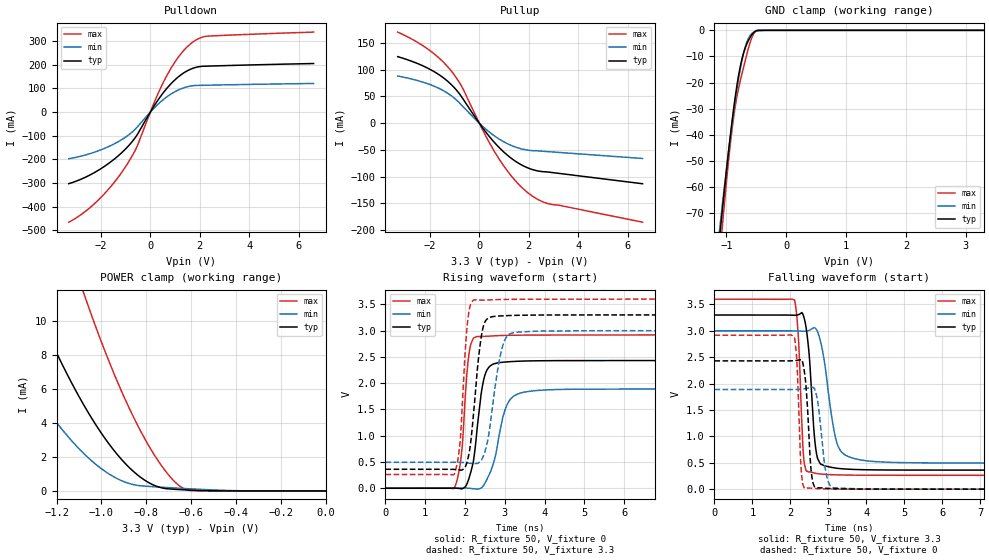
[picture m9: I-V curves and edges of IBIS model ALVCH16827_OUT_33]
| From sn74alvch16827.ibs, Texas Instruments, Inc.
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[Model]   ALVCH16827_OUT_33
Model_type  3-state
Enable   Active-Low
Vref =   0
Rref =   500
Cref =   50p
Vmeas =   1.5
| variable   typ   min   max
C_comp   3.97pF   3.54pF   4.17pF
| C_pullup   5.12pF   4.43pF   5.61pF
| C_pulldown   8.30pF   4.57pF   11.95pF
| C_tri-state   3.97pF   3.54pF   4.17pF
[Temperature Range]   40   100   -40
| Ambient temperature   25   85   -40
[Voltage range]   3.3   3   3.6
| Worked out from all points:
|   slope of the pulldown table from 0 to 0.495 V, typ, clamps not added: 6.36 ohm
|   slope of the pullup table from 0 to 0.495 V, typ, clamps not added: 16.5 ohm
|   GND clamp passes 1 mA (typ) near -0.55 V on its own axis
|   POWER clamp passes 1 mA (typ) near -0.84 V on its own axis
|   rising waveform, R_fixture 50, V_fixture 0: 20-80 % time 235ps typ, 343ps min, 166ps max; typ from 0 V to 2.43 V
|   falling waveform, R_fixture 50, V_fixture 3.3: 20-80 % time 167ps typ, 304ps min, 117ps max; typ from 3.3 V to 0.361 V
|   rising waveform, R_fixture 50, V_fixture 3.3: 20-80 % time 223ps typ, 290ps min, 155ps max; typ from 0.361 V to 3.3 V
|   falling waveform, R_fixture 50, V_fixture 0: 20-80 % time 119ps typ, 174ps min, 90.7ps max; typ from 2.43 V to 0 V
[GND Clamp]
| ALVCH16827_OUT_33
|   Voltage   I(typ)   I(min)   I(max)
-3.3V     -675.5mA   -611.9mA   -772mA
-1.12V    -80.81mA   -77.55mA   -88.84mA
-1.1V     -76.16mA   -73.37mA   -83.51mA
-1.075V   -70.43mA   -68.21mA   -76.96mA
-1.055V   -65.91mA   -64.14mA   -71.81mA
-905mV    -34.72mA   -35.65mA   -37.77mA
-845mV    -24.31mA   -25.69mA   -28.1mA
-780mV    -15.21mA   -16.34mA   -20.53mA
-655mV    -4.986mA   -4.361mA   -8.861mA
-575mV    -1.715mA   -1.195mA   -2.821mA
-510mV    -244.5uA   -419.5uA   -312.1uA
3.3V      1.222nA    1.002uA    51.57pA
[POWER Clamp]
| ALVCH16827_OUT_33
|   Voltage   I(typ)   I(min)   I(max)
-3.3V     106mA      74.09mA    151.6mA
-1.545V   19.46mA    11.49mA    33.45mA
-1.32V    11.68mA    6.284mA    22.02mA
-1.295V   10.9mA     5.78mA     20.85mA
-1.195V   7.991mA    3.942mA    16.37mA
-1.075V   4.975mA    2.155mA    11.49mA
-965mV    2.743mA    987.9uA    7.581mA
-860mV    1.177mA    378.6uA    4.425mA
-760mV    302.3uA    241.6uA    2.031mA
-660mV    86.32uA    163.9uA    380.1uA
-605mV    48.51uA    124.7uA    22.06uA
-48.03fV  1.222nA    59.96nA    62.94pA
[Pulldown]
| ALVCH16827_OUT_33
|   Voltage   I(typ)   I(min)   I(max)
-3.3V     -302.4mA   -196.9mA   -465.1mA
-2.73V    -280.1mA   -184.3mA   -427.4mA
-2.16V    -249.3mA   -165.8mA   -377mA
-1.61V    -210.9mA   -141.8mA   -315.8mA
-1.105V   -166.3mA   -112.9mA   -246.6mA
-565mV    -100.8mA   -67.07mA   -151.3mA
185mV     31.43mA    20.51mA    47.78mA
665mV     100mA      64.12mA    153.8mA
1.17V     151.9mA    95.01mA    237.4mA
1.67V     182.8mA    110.5mA    291.9mA
2.31V     194mA      113.5mA    320.7mA
6.6V      205mA      120.8mA    337.8mA
[Pullup]
| ALVCH16827_OUT_33
|   Voltage   I(typ)   I(min)   I(max)
-3.3V     124.6mA    88.26mA    170.5mA
-2.055V   102.2mA    73.29mA    137.8mA
-1.565V   88.69mA    63.61mA    119.2mA
-1.15V    73.01mA    51.93mA    98.57mA
-690mV    47.45mA    32.47mA    66.81mA
180mV     -11.59mA   -7.766mA   -16.76mA
755mV     -43.3mA    -28.29mA   -63.76mA
1.375V    -68.47mA   -43.2mA    -103.3mA
1.995V    -84.31mA   -50.62mA   -131.4mA
2.4V      -89.62mA   -51.95mA   -143.5mA
2.81V     -91.58mA   -53.32mA   -150.8mA
6.6V      -113.3mA   -66.05mA   -185.3mA
[Ramp]
| ALVCH16827_OUT_33
| variable   typ   min   max
dV/dt_r   1.47/2.46E-10   1.14/3.56E-10   1.76/1.73E-10
dV/dt_f   1.79/1.84E-10   1.54/3.17E-10   2.00/1.20E-10
R_load = 50
[Rising Waveform]
| ALVCH16827_OUT_33
R_fixture =   50
C_fixture =   0
L_fixture =   0
V_fixture =   0
V_fixture_min = 0
V_fixture_max = 0
|   Time   V(typ)   V(min)   V(max)
0s        334.5pV    1.078nV    249pV
1.725ns   3.449mV    326.4uV    -1.905mV
1.905ns   -10.46mV   2.905mV    619.5mV
2.105ns   206mV      -508.8uV   2.586V
2.305ns   1.149V     -17.32mV   2.889V
2.455ns   2.016V     43.54mV    2.891V
2.615ns   2.317V     274.4mV    2.897V
3.105ns   2.409V     1.659V     2.912V
3.995ns   2.429V     1.871V     2.917V
50ns      2.431V     1.889V     2.918V
[Falling Waveform]
| ALVCH16827_OUT_33
R_fixture =   50
C_fixture =   0
L_fixture =   0
V_fixture =   3.3
V_fixture_min = 3
V_fixture_max = 3.6
|   Time   V(typ)   V(min)   V(max)
0s        3.3V       3V         3.6V
2.11ns    3.295V     2.999V     3.585V
2.215ns   3.307V     2.997V     2.846V
2.37ns    3.228V     2.994V     486.5mV
2.5ns     2.53V      3.01V      327.7mV
2.66ns    828.5mV    3.05V      301.7mV
2.815ns   467.8mV    2.744V     285.9mV
3.265ns   393.4mV    806.3mV    270.2mV
4.265ns   365.1mV    520.8mV    263.7mV
50ns      361.2mV    493.5mV    262.9mV
[Rising Waveform]
| ALVCH16827_OUT_33
R_fixture =   50
C_fixture =   0
L_fixture =   0
V_fixture =   3.3
V_fixture_min = 3
V_fixture_max = 3.6
|   Time   V(typ)   V(min)   V(max)
0s        361.2mV    493.5mV    262.9mV
1.725ns   359.2mV    493.9mV    264mV
1.875ns   347.5mV    492.3mV    872.2mV
2.07ns    558.4mV    480.4mV    3.208V
2.23ns    1.56V      469.9mV    3.587V
2.375ns   2.707V     505.7mV    3.583V
2.5ns     3.168V     698.5mV    3.583V
2.95ns    3.284V     2.72V      3.594V
3.405ns   3.294V     2.977V     3.598V
50ns      3.3V       3V         3.6V
[Falling Waveform]
| ALVCH16827_OUT_33
R_fixture =   50
C_fixture =   0
L_fixture =   0
V_fixture =   0
V_fixture_min = 0
V_fixture_max = 0
|   Time   V(typ)   V(min)   V(max)
0s        2.431V     1.889V     2.918V
2.11ns    2.434V     1.888V     2.873V
2.18ns    2.442V     1.889V     2.315V
2.285ns   2.453V     1.894V     388.4mV
2.38ns    2.178V     1.903V     16.35mV
2.555ns   313.7mV    1.934V     17.97mV
2.71ns    23.42mV    1.713V     10.32mV
2.94ns    16.99mV    316.3mV    5.35mV
3.16ns    8.599mV    23.76mV    3.092mV
50ns      23.7nV     2.484nV    1.69nV
